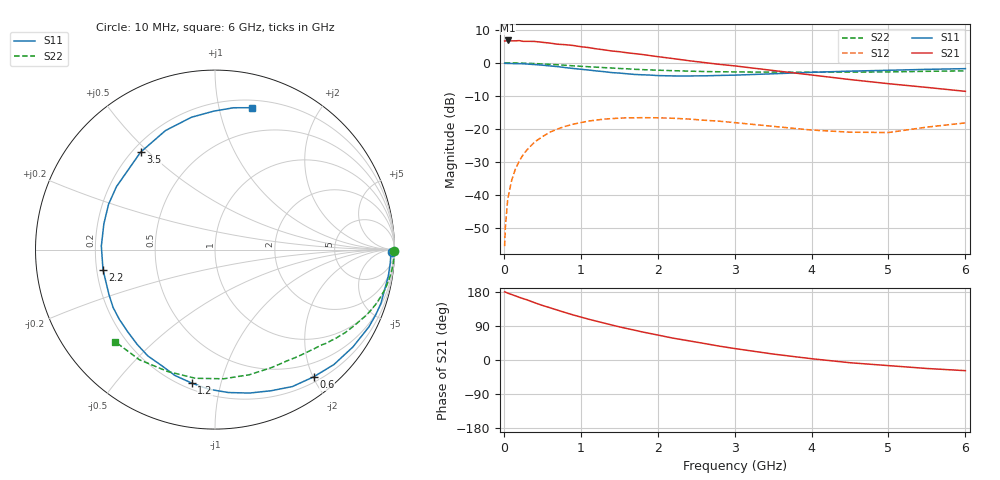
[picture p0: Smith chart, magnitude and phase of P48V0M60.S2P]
! SIEMENS Small Signal Semiconductors
! BFP182
! Si NPN RF Bipolar Junction Transistor in SOT143
! VCE = 8 V  IC = 0.6 mA
! Common Emitter S-Parameters:  March  1996
# GHz  S  MA  R  50
!  f  S11  S21  S12  S22
! GHz  MAG  ANG  MAG  ANG  MAG  ANG  MAG  ANG
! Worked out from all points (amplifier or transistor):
!   36 points, 10 MHz to 6 GHz, reference 50 ohm
!   highest |S21| = 6.8 dB at 50 MHz (marker M1)
!   |S21| within 3 dB of that: start of sweep to 1.351 GHz
!   unconditionally stable (mu >= 1): 2.882 GHz to end of sweep
!   at 250 MHz: K = 0.08, MSG = 17.2 dB, |S12| = -27.8 dB
!   at 1.4 GHz: K = 0.50, MSG = 10.2 dB, |S12| = -16.9 dB
!   at 6 GHz: K = 1.17, MAG = 2.3 dB, |S12| = -18.1 dB
!   S11 on the Smith chart (normalised r, x): 10 MHz: open; 600 MHz: 0.28, -2.01; 1.2 GHz: 0.24, -0.81; 2.2 GHz: 0.23, -0.08; 3.5 GHz: 0.23, +0.47; 6 GHz: 0.27, +1.26
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0.01  0.9846 -0.7  2.138 179.6  0.0017 82.4  0.9985 -0.3
0.02  0.9802 -1.6  2.141 179.3  0.0033 93.1  0.9966 -0.6
0.05  0.9795 -4.4  2.177 176.4  0.0086 88.7  0.9978 -1.6
0.1  0.9768 -8.7  2.145 172.9  0.0165 84.3  0.9972 -3.2
0.15  0.971 -13.5  2.149 169.3  0.0248 80.8  0.995 -4.9
0.2  0.9718 -17.9  2.166 165.5  0.0328 78.3  0.9925 -6.5
0.25  0.9665 -22.1  2.112 162.0  0.0407 75.8  0.9881 -8.2
0.4  0.9406 -35.2  2.105 151.2  0.0635 67.1  0.9746 -12.7
0.6  0.8971 -52.2  1.985 137.9  0.0897 56.3  0.9483 -18.4
0.9  0.822 -76.5  1.829 119.0  0.1184 41.9  0.9011 -25.9
1.1  0.7789 -92.5  1.701 107.8  0.1318 33.2  0.8727 -30.4
1.2  0.7547 -99.9  1.627 102.7  0.1364 29.2  0.8598 -32.6
1.6  0.6833 -129.4  1.42 83.0  0.1478 16.1  0.8127 -39.8
1.8  0.6596 -144.0  1.336 74.0  0.1483 11.0  0.7894 -43.2
2.2  0.634 -169.9  1.159 57.7  0.1453 1.4  0.7609 -50.0
2.8  0.6446 156.9  0.949 36.6  0.1313 -8.4  0.7329 -60.5
3.5  0.683 127.4  0.766 15.7  0.1097 -12.9  0.723 -74.7
4  0.7183 112.6  0.655 3.4  0.0965 -9.7  0.7214 -86.2
4.5  0.749 100.1  0.559 -7.2  0.0896 -3.3  0.7252 -98.7
5  0.7715 90.5  0.484 -14.8  0.0885 9.2  0.7286 -111.3
5.5  0.7969 82.6  0.425 -22.4  0.1069 14.5  0.7444 -124.5
6  0.8165 75.5  0.371 -28.1  0.1238 15.6  0.7567 -137.3
